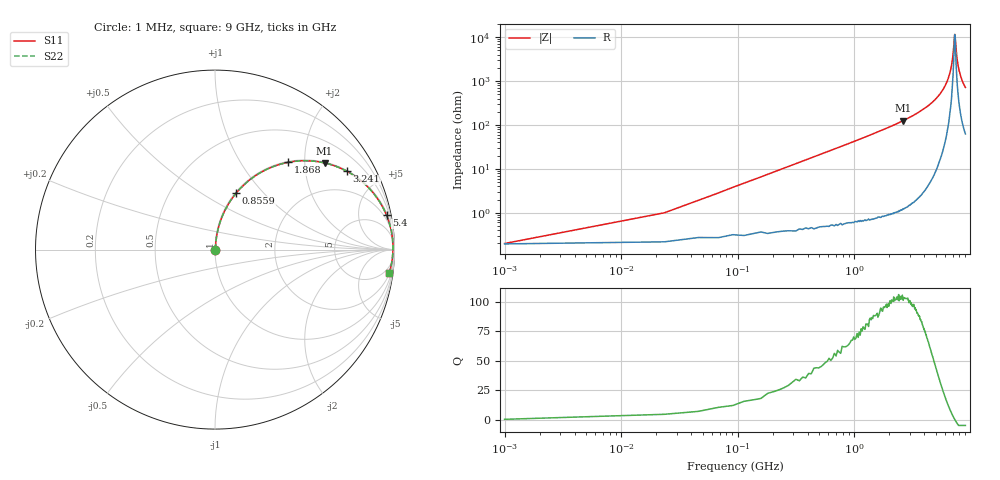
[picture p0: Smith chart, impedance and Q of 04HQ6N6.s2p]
! Coilcraft 0403HQ-6N6 Chip Inductor
! 13 February 2004
# MHZ S MA R 50
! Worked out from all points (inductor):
!   401 points, 1 MHz to 9 GHz, reference 50 ohm
!   read as one part in series: L = 6.57 nH near 45.99 MHz
!   highest Q = 103 at 2.633 GHz (marker M1), where L = 7.58 nH
!   self-resonance near 7.29 GHz
!   S11 on the Smith chart (normalised r, x): 1 MHz: 1.00, +0.00; 855.9 MHz: 1.01, +0.72; 1.868 GHz: 1.02, +1.66; 3.241 GHz: 1.03, +3.35; 5.4 GHz: 1.27, +9.88; 9 GHz: 2, -14
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1  0.001932 12.3  0.998 -0.0  0.998 -0.0  0.001932 12.3
68.492  0.028 82.7  0.997 -1.6  0.997 -1.6  0.028 82.7
90.99  0.038 83.3  0.996 -2.2  0.996 -2.2  0.038 83.3
203.477  0.084 82.7  0.993 -4.8  0.993 -4.8  0.084 82.7
450.95  0.184 78.0  0.979 -10.6  0.979 -10.6  0.184 78.0
855.905  0.337 69.4  0.936 -19.7  0.936 -19.7  0.337 69.4
1508.332  0.544 56.4  0.833 -33.0  0.833 -33.0  0.544 56.4
1868.292  0.635 50.0  0.766 -39.4  0.766 -39.4  0.635 50.0
2633.207  0.778 38.3  0.62 -51.1  0.62 -51.1  0.778 38.3
3015.665  0.83 33.4  0.55 -56.0  0.55 -56.0  0.83 33.4
3240.64  0.855 30.7  0.511 -58.7  0.511 -58.7  0.855 30.7
4500.5  0.944 18.3  0.314 -70.8  0.314 -70.8  0.944 18.3
5400.4  0.975 11.4  0.197 -76.9  0.197 -76.9  0.975 11.4
6007.833  0.985 7.3  0.128 -79.7  0.128 -79.7  0.985 7.3
6795.245  0.991 2.7  0.048 -78.0  0.048 -78.0  0.991 2.7
7020.22  0.992 1.5  0.027 -71.2  0.027 -71.2  0.992 1.5
7290.19  0.991 0.1  0.008582 -7.5  0.008582 -7.5  0.991 0.1
7357.683  0.991 -0.3  0.009921 29.3  0.009921 29.3  0.991 -0.3
7515.165  0.991 -1.1  0.021 63.5  0.021 63.5  0.991 -1.1
7762.638  0.99 -2.3  0.041 74.5  0.041 74.5  0.99 -2.3
8032.608  0.988 -3.6  0.063 77.4  0.063 77.4  0.988 -3.6
9000  0.979 -7.8  0.136 77.2  0.136 77.2  0.979 -7.8
